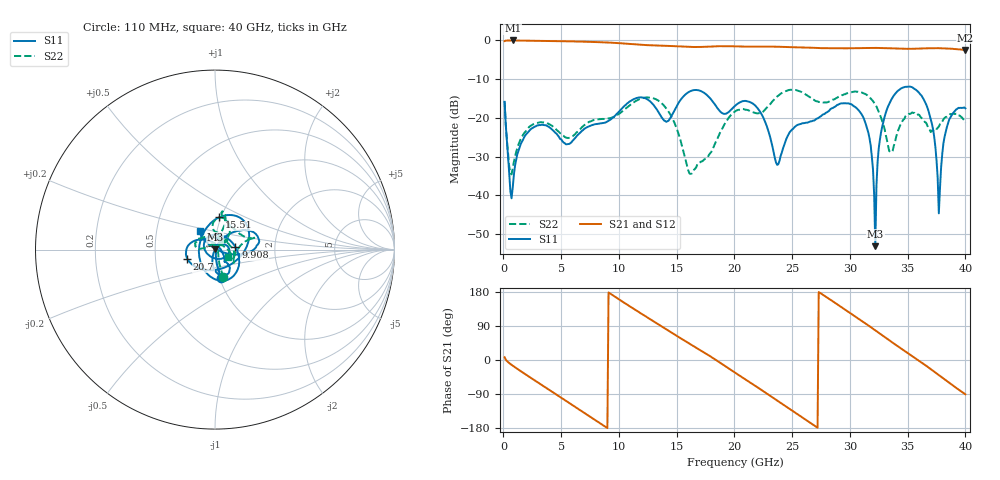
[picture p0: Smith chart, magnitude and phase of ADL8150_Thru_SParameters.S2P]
! Analog Devices, Inc.
! Device:	ADL8150ACPZN - THRU
! Description:	"GaAs, HBT, MMIC, Low Phase Noise Amplifier, 6 GHz to 14 GHz"
! Conditions:	Pin = -20 dBm
!		Operating Temperature = +25 C (at package bottom)
! Measurement used thru-cal line of SN#19.
! Frequency (GHz)	S11_Mag (dB)	S11_Phase (deg)	S21_Mag (dB)	S21_Phase (deg)	S12_Mag (dB)	S12_Phase (deg)	S22_Mag (dB)	S22_Phase (deg)
#  GHZ  S  DB  R 50
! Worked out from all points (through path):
!   400 points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, 110 MHz to 40 GHz, reference 50 ohm
!   highest |S21| = -0.14 dB at 809.8 MHz (marker M1); lowest = -2.6 dB at 40 GHz (marker M2)
!   group delay of S21, straight-line fit = 55.8 ps
!   lowest |S11| = -53.1 dB at 32.2 GHz (marker M3), VSWR 1.00, Z = 50.1 + j0.211 ohm
!   |S11| at or under -10 dB: start of sweep to end of sweep
!   |S22| runs from -34.6 to -12.8 dB; largest |S21 - S12| = 0.0038
!   S11 on the Smith chart (normalised r, x): 110 MHz: 1.01, -0.33; 9.908 GHz: 1.26, +0.03; 15.51 GHz: 0.98, +0.37; 20.7 GHz: 0.73, -0.08; 40 GHz: 0.83, +0.17
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0.109975  -15.93 -78.3  -0.29 7.2  -0.28 7.2  -15.82 -73.5
0.8098  -38.09 26.3  -0.14 -15.0  -0.14 -14.9  -33.10 24.6
2.4094  -22.88 16.3  -0.22 -47.7  -0.21 -47.7  -22.02 46.1
6.8083  -23.39 156.5  -0.44 -135.6  -0.44 -135.6  -22.45 83.4
9.907525  -18.80 6.3  -0.81 162.1  -0.81 162.2  -19.23 94.2
13.40665  -18.45 -125.1  -1.44 94.6  -1.44 94.7  -15.60 62.7
15.50613  -14.82 82.3  -1.74 54.4  -1.73 54.4  -27.75 43.5
16.30592  -13.05 56.4  -1.82 39.7  -1.82 39.7  -34.39 95.9
20.10497  -16.85 -138.0  -1.66 -34.4  -1.66 -34.4  -18.29 -30.2
20.70482  -15.76 -161.5  -1.70 -46.3  -1.70 -46.2  -17.79 -35.2
23.70407  -32.15 50.3  -1.75 -107.1  -1.75 -107.0  -14.56 16.0
26.70332  -20.93 -50.3  -2.01 -168.5  -2.02 -168.4  -15.10 24.9
31.10222  -19.57 -93.8  -2.10 101.7  -2.10 101.8  -13.62 75.6
31.90203  -30.07 -109.9  -2.06 84.7  -2.07 84.7  -15.36 70.2
32.20195  -53.07 71.2  -2.05 78.2  -2.07 78.3  -16.68 68.8
32.50187  -27.82 61.6  -2.07 71.7  -2.06 71.8  -18.52 69.3
33.40165  -16.52 41.9  -2.15 52.1  -2.13 52.2  -28.56 102.3
36.60085  -16.58 -10.5  -2.16 -15.1  -2.15 -15.0  -21.32 118.8
37.30067  -24.95 -18.5  -2.13 -30.9  -2.12 -30.7  -23.44 61.5
37.70058  -44.63 50.0  -2.12 -39.8  -2.12 -39.8  -22.31 30.2
38.4004  -22.40 137.7  -2.21 -55.6  -2.20 -55.7  -19.75 -1.7
40  -17.61 129.5  -2.62 -90.6  -2.61 -90.6  -21.30 -30.4
